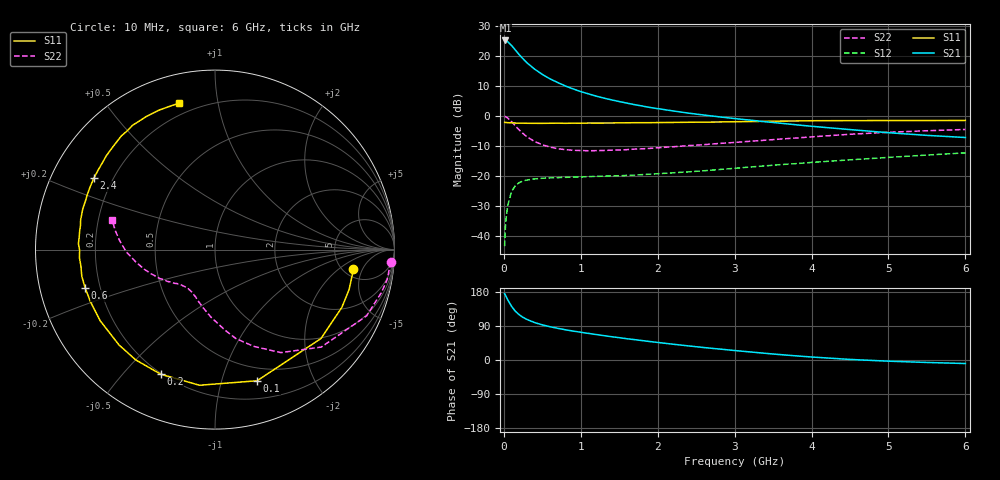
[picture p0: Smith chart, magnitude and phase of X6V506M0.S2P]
! SIEMENS Small Signal Semiconductors
! BFP193W
! Si NPN RF Bipolar Junction Transistor in SOT343
! VCE = 0.5 V  IC = 6 mA
! Common Emitter S-Parameters:  April 1994
# GHz  S  MA  R  50
!  f  S11  S21  S12  S22
! GHz  MAG  ANG  MAG  ANG  MAG  ANG  MAG  ANG
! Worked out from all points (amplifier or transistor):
!   40 points, 10 MHz to 6 GHz, reference 50 ohm
!   highest |S21| = 25.1 dB at 20 MHz (marker M1)
!   |S21| within 3 dB of that: start of sweep to 143.4 MHz
!   unconditionally stable (mu >= 1): 1.412 GHz to end of sweep
!   at 200 MHz: K = 0.17, MSG = 21.3 dB, |S12| = -22.2 dB
!   at 1.5 GHz: K = 1.04, MAG = 11.2 dB, |S12| = -19.9 dB
!   at 6 GHz: K = 1.11, MAG = 0.5 dB, |S12| = -12.3 dB
!   S11 on the Smith chart (normalised r, x): 10 MHz: 6.11, -3.41; 100 MHz: 0.37, -1.31; 200 MHz: 0.20, -0.64; 600 MHz: 0.14, -0.14; 2.4 GHz: 0.13, +0.27; 6 GHz: 0.14, +0.78
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0.01  0.7792 -8.1  17.99 174.9  0.0068 85.7  0.9816 -4.0
0.02  0.7796 -16.6  18 171.4  0.0136 80.8  0.9736 -9.9
0.03  0.7767 -24.5  17.77 167.2  0.02 78.1  0.9578 -14.4
0.05  0.7708 -40.0  17.14 158.9  0.0322 70.4  0.922 -23.6
0.1  0.7674 -72.2  14.84 141.8  0.0551 55.1  0.8035 -42.5
0.15  0.7607 -96.5  12.45 128.5  0.0694 44.1  0.6814 -57.4
0.2  0.7571 -113.6  10.42 119.4  0.0776 36.7  0.5814 -68.1
0.25  0.7568 -125.7  8.9 112.4  0.0827 31.5  0.5091 -76.8
0.3  0.7539 -135.2  7.669 107.0  0.0857 28.1  0.449 -83.3
0.4  0.7525 -148.2  6 98.8  0.0893 23.6  0.3751 -93.7
0.5  0.7521 -157.0  4.902 92.7  0.0918 21.3  0.3311 -101.4
0.6  0.7544 -163.5  4.134 87.8  0.093 19.7  0.303 -107.7
0.8  0.7528 -172.9  3.148 79.8  0.0951 19.0  0.2744 -116.5
1.1  0.7616 177.5  2.327 70.2  0.0977 19.6  0.2629 -125.2
1.3  0.7612 172.0  1.979 64.3  0.0993 20.8  0.2661 -129.4
1.6  0.7681 165.1  1.631 56.1  0.1024 23.3  0.2745 -134.5
2.2  0.7787 153.2  1.21 41.7  0.113 28.0  0.3065 -143.8
2.4  0.7835 149.5  1.112 37.2  0.1172 29.3  0.3204 -146.5
3.2  0.8053 135.8  0.851 21.3  0.141 32.8  0.3782 -158.8
4.5  0.8344 117.3  0.592 1.5  0.1857 31.6  0.4947 -178.6
5.5  0.8372 107.9  0.474 -6.5  0.223 28.0  0.5662 169.1
6  0.8401 103.7  0.437 -9.3  0.2427 26.0  0.5951 164.1
